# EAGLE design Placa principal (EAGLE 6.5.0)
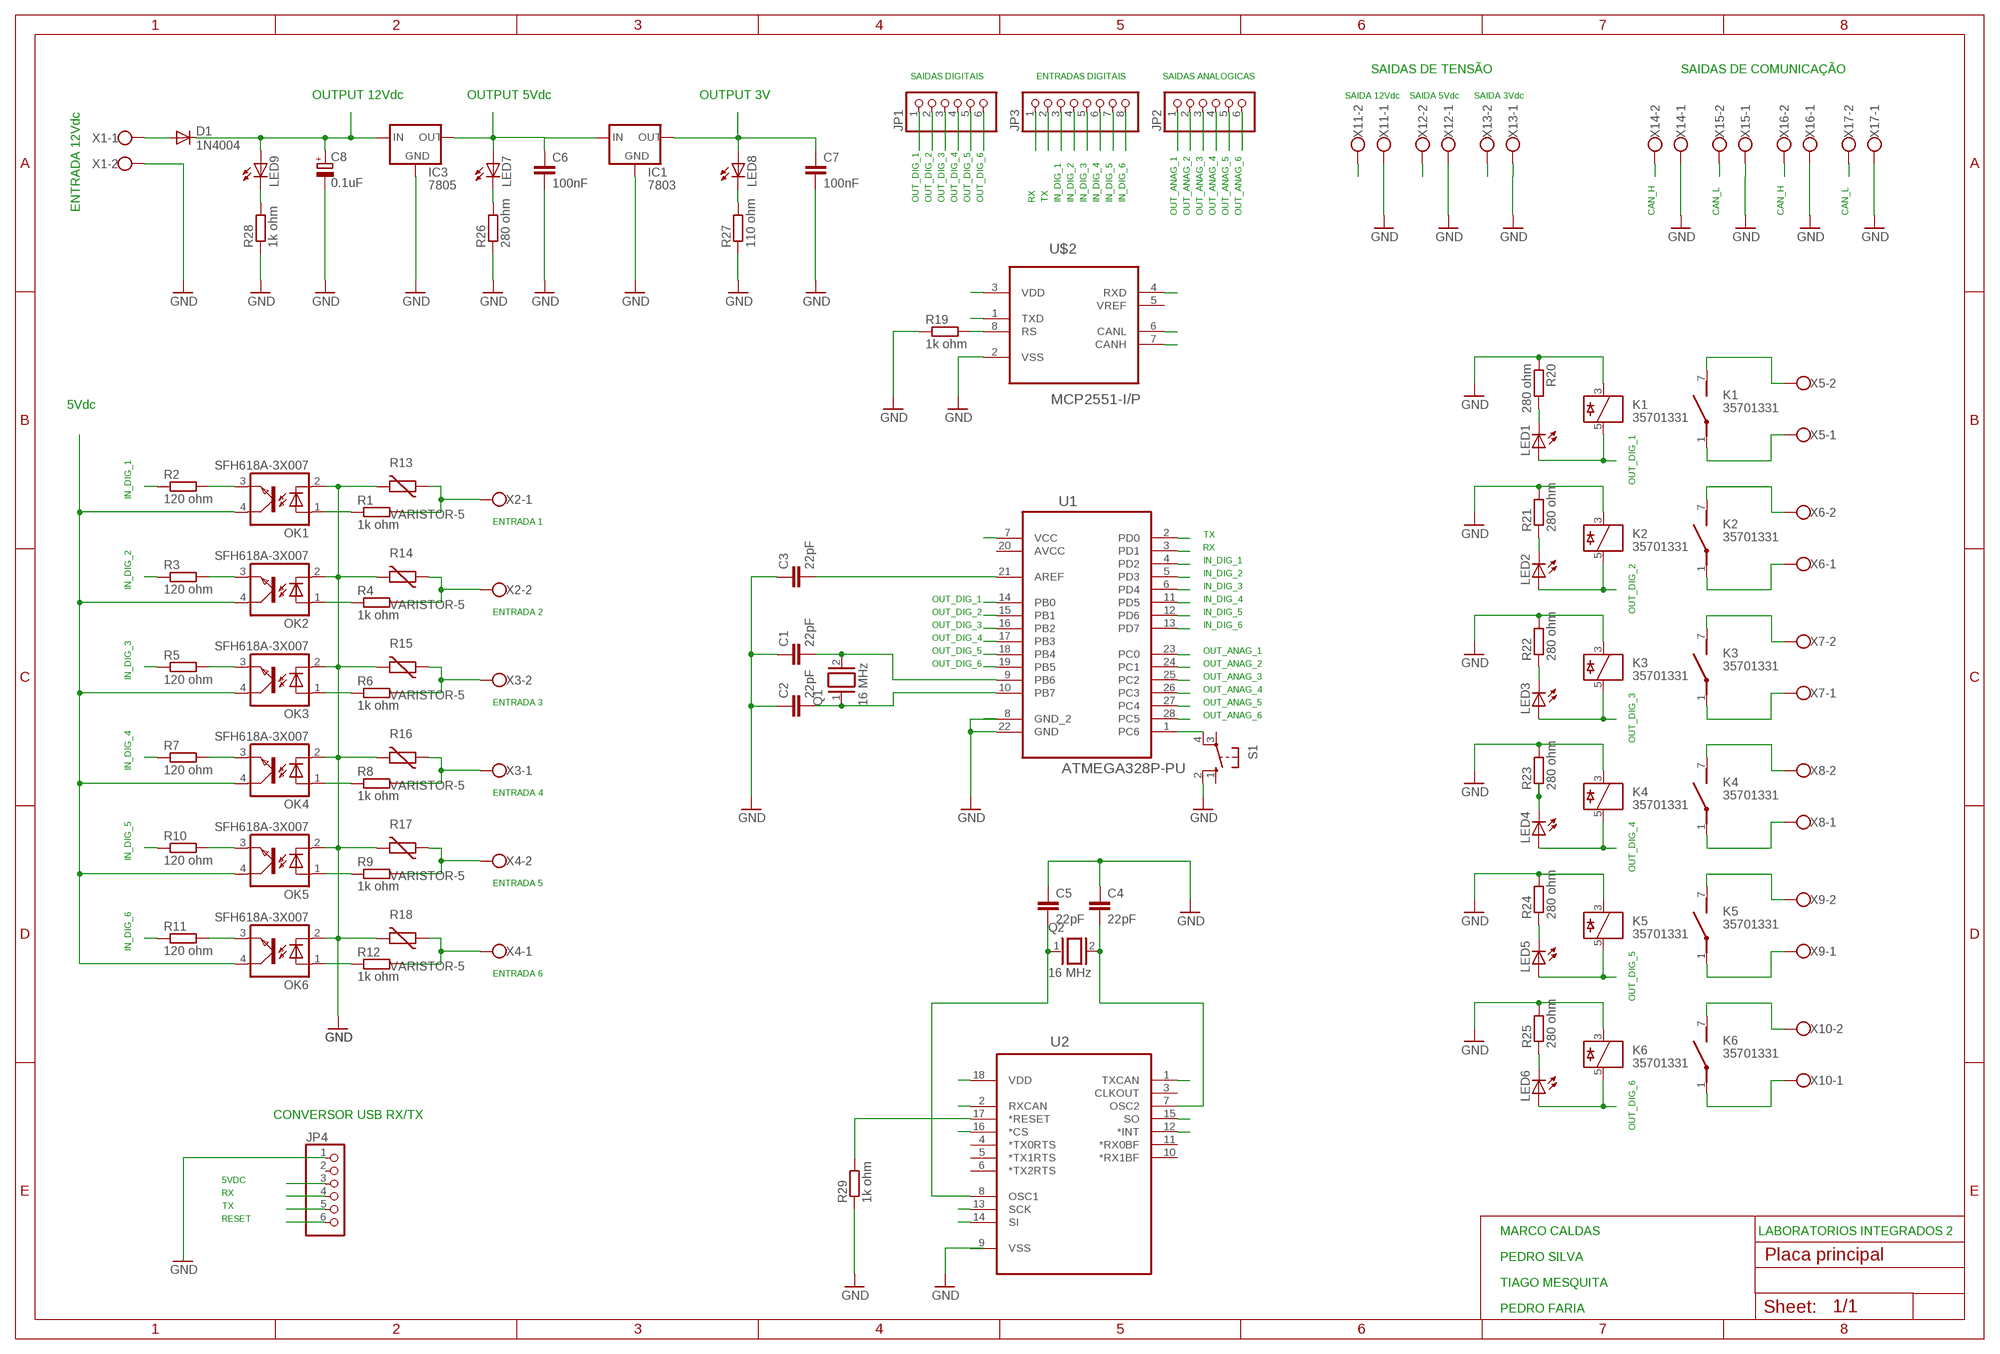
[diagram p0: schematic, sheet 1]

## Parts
C1  22pF  C-EU050-025X075  [C050-025X075]
C2  22pF  C-EU050-025X075  [C050-025X075]
C3  22pF  C-EU050-025X075  [C050-025X075]
C4  22pF  C-EU050-025X075  [C050-025X075]
C5  22pF  C-EU050-025X075  [C050-025X075]
C6  100nF  C-EU050-025X075  [C050-025X075]
C7  100nF  C-EU050-025X075  [C050-025X075]
C8  0.1uF  CPOL-EUE2.5-7  [E2,5-7]
D1  1N4004  [DO41-10]
IC1  7803  78XXS  [78XXS]
IC3  7805  78XXS  [78XXS]
JP1  PINHD-1X6  [1X06]
JP2  PINHD-1X6  [1X06]
JP3  PINHD-1X8  [1X08]
JP4  PINHD-1X6  [1X06]
K1  35701331  [REED]
K2  35701331  [REED]
K3  35701331  [REED]
K4  35701331  [REED]
K5  35701331  [REED]
K6  35701331  [REED]
LED1  LED5MM  [LED5MM]
LED2  LED5MM  [LED5MM]
LED3  LED5MM  [LED5MM]
LED4  LED5MM  [LED5MM]
LED5  LED5MM  [LED5MM]
LED6  LED5MM  [LED5MM]
LED7  LED5MM  [LED5MM]
LED8  LED5MM  [LED5MM]
LED9  LED5MM  [LED5MM]
OK1  SFH618A-3X007  [SMD4-7]
OK2  SFH618A-3X007  [SMD4-7]
OK3  SFH618A-3X007  [SMD4-7]
OK4  SFH618A-3X007  [SMD4-7]
OK5  SFH618A-3X007  [SMD4-7]
OK6  SFH618A-3X007  [SMD4-7]
Q1  16 MHz  XTAL/S  [QS]
Q2  16 MHz  XTAL/S  [QS]
R1  1k ohm  R-EU_0207/10  [0207/10]
R2  120 ohm  R-EU_0207/10  [0207/10]
R3  120 ohm  R-EU_0207/10  [0207/10]
R4  1k ohm  R-EU_0207/10  [0207/10]
R5  120 ohm  R-EU_0207/10  [0207/10]
R6  1k ohm  R-EU_0207/10  [0207/10]
R7  120 ohm  R-EU_0207/10  [0207/10]
R8  1k ohm  R-EU_0207/10  [0207/10]
R9  1k ohm  R-EU_0207/10  [0207/10]
R10  120 ohm  R-EU_0207/10  [0207/10]
R11  120 ohm  R-EU_0207/10  [0207/10]
R12  1k ohm  R-EU_0207/10  [0207/10]
R13  VARISTOR-5  [R-5]
R14  VARISTOR-5  [R-5]
R15  VARISTOR-5  [R-5]
R16  VARISTOR-5  [R-5]
R17  VARISTOR-5  [R-5]
R18  VARISTOR-5  [R-5]
R19  1k ohm  R-EU_0207/10  [0207/10]
R20  280 ohm  R-EU_0207/10  [0207/10]
R21  280 ohm  R-EU_0207/10  [0207/10]
R22  280 ohm  R-EU_0207/10  [0207/10]
R23  280 ohm  R-EU_0207/10  [0207/10]
R24  280 ohm  R-EU_0207/10  [0207/10]
R25  280 ohm  R-EU_0207/10  [0207/10]
R26  280 ohm  R-EU_0207/10  [0207/10]
R27  110 ohm  R-EU_0207/10  [0207/10]
R28  1k ohm  R-EU_0207/10  [0207/10]
R29  1k ohm  R-EU_0207/10  [0207/10]
S1  10-XX  [B3F-10XX]
U1  ATMEGA328P-PU  [DIP254P762X457-28]
U2  MCP2510-I/P.  [DIP254P762X533-18P]
U$2  MCP2551-I/P  [DIP254P762X432-8]
X1  W237-102  [W237-102]
X2  W237-102  [W237-102]
X3  W237-102  [W237-102]
X4  W237-102  [W237-102]
X5  W237-102  [W237-102]
X6  W237-102  [W237-102]
X7  W237-102  [W237-102]
X8  W237-102  [W237-102]
X9  W237-102  [W237-102]
X10  W237-102  [W237-102]
X11  W237-102  [W237-102]
X12  W237-102  [W237-102]
X13  W237-102  [W237-102]
X14  W237-102  [W237-102]
X15  W237-102  [W237-102]
X16  W237-102  [W237-102]
X17  W237-102  [W237-102]

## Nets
3VDC: C7.1 IC1.OUT LED8.A X13.2
5VDC: C6.1 IC1.IN IC3.OUT JP4.3 LED7.A OK1.4(COL) OK2.4(COL) OK3.4(COL) OK4.4(COL) OK5.4(COL) OK6.4(COL) U1.7(VCC) U2.18(VDD) U$2.3(VDD) X12.2
12VDC: C8.+ D1.C IC3.IN LED9.A X11.2
CAN_H: U$2.7(CANH) X14.2 X16.2
CAN_L: U$2.6(CANL) X15.2 X17.2
CAN_RX: U2.1(TXCAN) U$2.4(RXD)
CAN_TX: U2.2(RXCAN) U$2.1(TXD)
GND: C1.1 C2.1 C3.1 C4.1 C5.1 C6.2 C7.2 C8.- IC1.GND IC3.GND JP4.1 K1.3 K2.3 K3.3 K4.3 K5.3 K6.3 OK1.2(C) OK2.2(C) OK3.2(C) OK4.2(C) OK5.2(C) OK6.2(C) R13.2 R14.2 R15.2 R16.2 R17.2 R18.2 R19.1 R20.1 R21.2 R22.2 R23.2 R24.2 R25.2 R26.1 R27.1 R28.1 R29.1 S1.2(S1) U1.8(GND_2) U1.22(GND) U$2.2(VSS) X1.2 X11.1 X12.1 X14.1 X16.1 X17.1
IN_DIG_1: JP3.3 R2.1 U1.4(PD2) U2.12(*INT)
IN_DIG_2: JP3.4 R3.1 U1.5(PD3)
IN_DIG_3: JP3.5 R5.1 U1.6(PD4)
IN_DIG_4: JP3.6 R7.1 U1.11(PD5)
IN_DIG_5: JP3.7 R10.1 U1.12(PD6)
IN_DIG_6: JP3.8 R11.1 U1.13(PD7)
N$1: OK1.3(EMIT) R2.2
N$2: OK1.1(A) R1.1
N$3: X15.1
N$4: K1.7(2:S) X5.2
N$5: OK2.1(A) R4.1
N$6: OK3.1(A) R6.1
N$7: OK4.1(A) R8.1
N$8: OK2.3(EMIT) R3.2
N$9: OK3.3(EMIT) R5.2
N$10: OK4.3(EMIT) R7.2
N$11: OK5.3(EMIT) R10.2
N$12: OK6.3(EMIT) R11.2
N$13: K1.1(2:P) X5.1
N$14: R1.2 R13.1 X2.1
N$15: OK6.1(A) R12.1
N$16: OK5.1(A) R9.1
N$17: R4.2 R14.1 X2.2
N$18: R6.2 R15.1 X3.2
N$19: R8.2 R16.1 X3.1
N$20: R9.2 R17.1 X4.2
N$21: R12.2 R18.1 X4.1
N$22: LED2.K(C) R21.1
N$24: LED1.K(C) R20.2
N$25: C1.2 Q1.2 U1.9(PB6)
N$26: C2.2 Q1.1 U1.10(PB7)
N$27: K2.7(2:S) X6.2
N$28: C3.2 U1.21(AREF)
N$30: LED3.K(C) R22.1
N$31: R19.2 U$2.8(RS)
N$32: D1.A X1.1
N$33: C4.2 Q2.2 U2.7(OSC2)
N$34: C5.2 Q2.1 U2.8(OSC1)
N$35: R29.2 U2.17(*RESET)
N$38: K2.1(2:P) X6.1
N$39: LED4.K(C) R23.1
N$41: K3.7(2:S) X7.2
N$42: LED5.K(C) R24.1
N$43: LED7.K(C) R26.2
N$44: K3.1(2:P) X7.1
N$45: LED6.K(C) R25.1
N$46: LED8.K(C) R27.2
N$47: K4.7(2:S) X8.2
N$48: LED9.K(C) R28.2
N$50: K4.1(2:P) X8.1
N$51: K5.7(2:S) X9.2
N$52: K5.1(2:P) X9.1
N$53: K6.7(2:S) X10.2
N$54: K6.1(2:P) X10.1
N$57: X13.1
OUT_ANAG_1: JP2.1 U1.23(PC0)
OUT_ANAG_2: JP2.2 U1.24(PC1)
OUT_ANAG_3: JP2.3 U1.25(PC2)
OUT_ANAG_4: JP2.4 U1.26(PC3)
OUT_ANAG_5: JP2.5 U1.27(PC4)
OUT_ANAG_6: JP2.6 U1.28(PC5)
OUT_DIG_1: JP1.1 K1.5 LED1.A U1.14(PB0)
OUT_DIG_2: JP1.2 K2.5 LED2.A U1.15(PB1)
OUT_DIG_3: JP1.3 K3.5 LED3.A U1.16(PB2) U2.16(*CS)
OUT_DIG_4: JP1.4 K4.5 LED4.A U1.17(PB3) U2.14(SI)
OUT_DIG_5: JP1.5 K5.5 LED5.A U1.18(PB4) U2.15(SO)
OUT_DIG_6: JP1.6 K6.5 LED6.A U1.19(PB5) U2.13(SCK)
RESET: JP4.6 S1.4(P1) U1.1(PC6)
RX: JP3.1 JP4.4 U1.3(PD1)
TX: JP3.2 JP4.5 U1.2(PD0)
Unconnected: JP4.2 S1.1(S) S1.3(P) U2.3(CLKOUT) U2.4(*TX0RTS) U2.5(*TX1RTS) U2.6(*TX2RTS) U2.10(*RX1BF) U2.11(*RX0BF) U$2.5(VREF)

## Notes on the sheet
- SAIDAS DIGITAIS | ENTRADAS DIGITAIS | SAIDAS ANALOGICAS | SAIDAS DE TENSÃO | SAIDAS DE COMUNICAÇÃO
- OUTPUT 12Vdc | OUTPUT 5Vdc | OUTPUT 3V | SAIDA 12Vdc | SAIDA 5Vdc | SAIDA 3Vdc
- OUT_DIG_1 | OUT_DIG_2 | OUT_DIG_3 | OUT_DIG_4 | OUT_DIG_5 | OUT_DIG_6 | RX | TX | IN_DIG_1 | IN_DIG_2 | IN_DIG_3 | IN_DIG_4 | IN_DIG_5 | IN_DIG_6
- ENTRADA 12Vdc | OUT_ANAG_1 | OUT_ANAG_2 | OUT_ANAG_3 | OUT_ANAG_4 | OUT_ANAG_5 | OUT_ANAG_6 | CAN_H | CAN_L | CAN_H | CAN_L
- 5Vdc
- OUT_DIG_1
- IN_DIG_1
- ENTRADA 1
- TX
- RX
- IN_DIG_1 | OUT_DIG_2
- IN_DIG_2
- IN_DIG_2 | IN_DIG_3
- OUT_DIG_1 | IN_DIG_4
- ENTRADA 2 | OUT_DIG_2 | IN_DIG_5
- OUT_DIG_3 | IN_DIG_6
- OUT_DIG_4
- OUT_DIG_5 | OUT_ANAG_1
- OUT_DIG_6 | OUT_ANAG_2
- IN_DIG_3 | OUT_ANAG_3
- OUT_ANAG_4 | OUT_DIG_3
- ENTRADA 3 | OUT_ANAG_5
- OUT_ANAG_6
- IN_DIG_4
- ENTRADA 4
- OUT_DIG_4
- IN_DIG_5
- ENTRADA 5
- IN_DIG_6 | OUT_DIG_5
- ENTRADA 6
- OUT_DIG_6
- CONVERSOR USB RX/TX
- 5VDC
- RX
- TX
- RESET
- MARCO CALDAS | LABORATORIOS INTEGRADOS 2
- PEDRO SILVA
- TIAGO MESQUITA
- PEDRO FARIA

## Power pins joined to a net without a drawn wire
AVCC: U1.20(AVCC)
VSS: U2.9(VSS)

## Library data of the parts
C1-C7 = rcl:C-EU: CAPACITOR, European symbol
C8 = rcl:CPOL-EU: POLARIZED CAPACITOR, European symbol
D1 = diode:1N4004: DIODE
IC1 IC3 = v-reg:78XXS: VOLTAGE REGULATOR
JP1 JP2 JP4 = pinhead:PINHD-1X6: PIN HEADER
JP3 = pinhead:PINHD-1X8: PIN HEADER
K1-K6 = relay:35701331: RELAY reed, 1 x norm. open with polarity; OC_FARNELL: unknown; OC_NEWARK: unknown
LED1-LED9 = led:LED: LED
OK1-OK6 = optocoupler:SFH618?*: Optocoupler, Phototransistor Output, Low Input Current Source: Data sheet; OC_FARNELL: unknown; OC_NEWARK: unknown
Q1 Q2 = special:XTAL/S: CRYSTAL
R1-R12 R19-R29 = rcl:R-EU_: RESISTOR, European symbol
R13-R18 = varistor:VARISTOR: VARISTOR
S1 = switch-omron:10-XX: OMRON SWITCH; MPN: B3F-1000; OC_FARNELL: 176432; OC_NEWARK: 36M3542
U1 = atmega 328:ATMEGA328P-PU: 8-bit Microcontroller with In-System Programmable Flash; MPN: ATMEGA328P-PU; OC_FARNELL: 1715487; OC_NEWARK: 15R0268; PACKAGE: PDIP-28; SUPPLIER: Atmel
U2 = MCP2510:MCP2510-I/P.: IC, Stand-Alone CAN Controller with SPI Interface, DIP-18; MPN: MCP2510-I/P.; OC_FARNELL: 9758534; OC_NEWARK: 12C1807; PACKAGE: DIP-18; SUPPLIER: Microchip
U$2 = MCP:MCP2551-I/P: High-Speed CAN Transceiver; DESCRIPTION: CAN CTRL; MPN: MCP2551-I/P; OC_FARNELL: 1292240; OC_NEWARK: 61K2947; PACKAGE: PDIP-8; SUPPLIER: Microchip
X1-X17 = con-wago-500:W237-102: WAGO SCREW CLAMP; MPN: 237-102; OC_FARNELL: unknown; OC_NEWARK: 70K9898

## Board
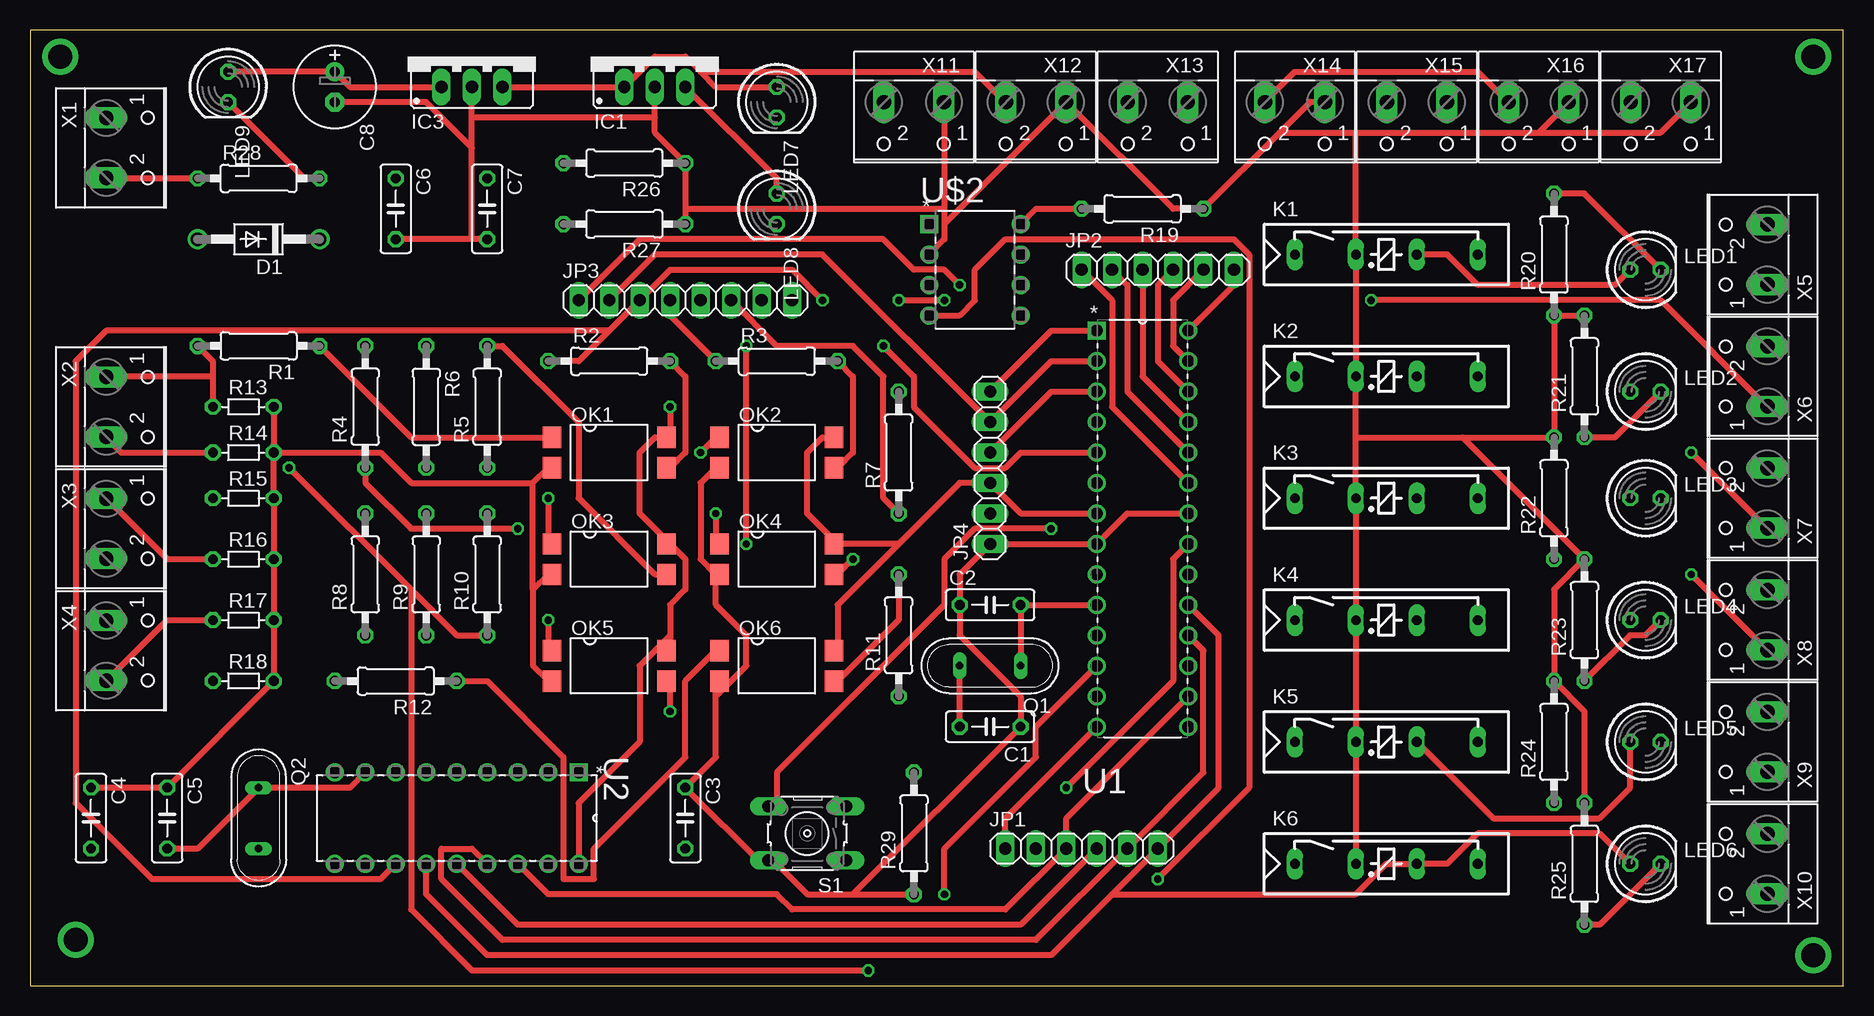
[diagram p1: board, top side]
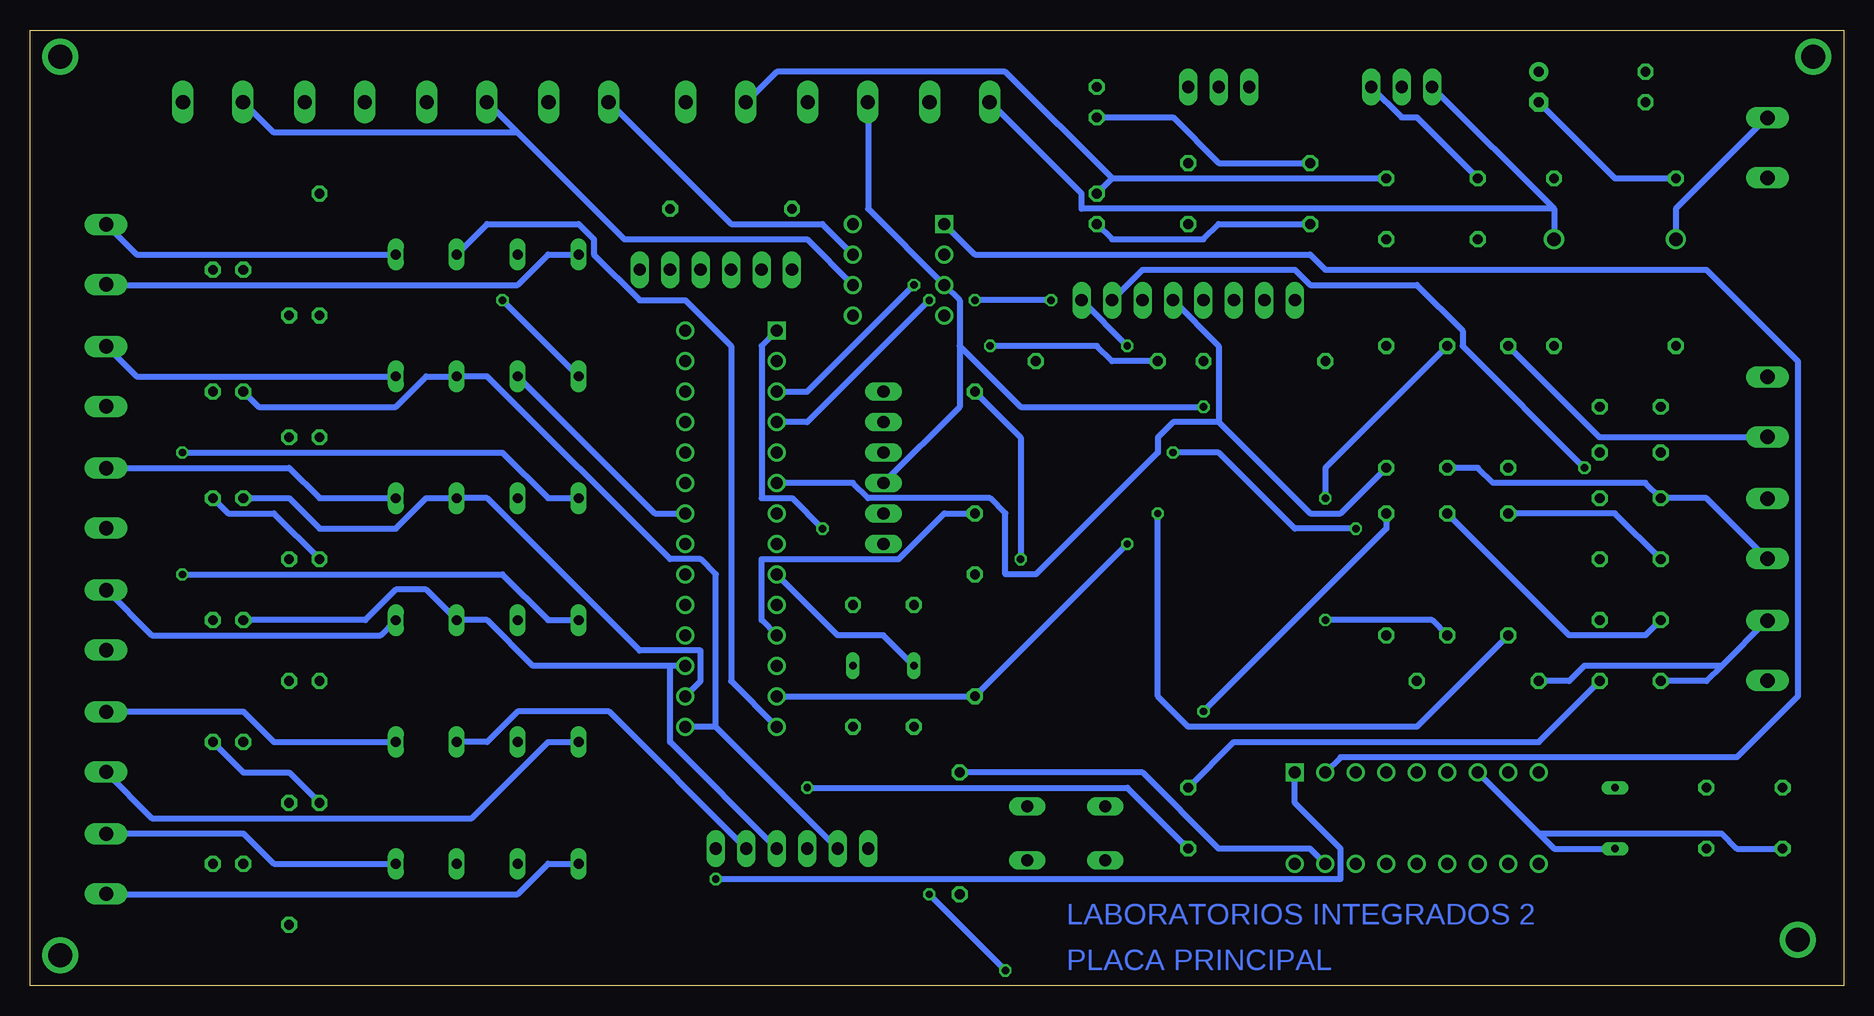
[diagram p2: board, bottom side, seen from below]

Size 151.13 x 79.68 mm. Coordinates in mm from the lower left corner, seen from the top.
Outline: 151.11,0 151.11,79.68 0,79.68 0,0 151.13,0
Copper layers (1*16): Top 0.035mm / dielectric 1.5mm / Bottom 0.035mm
Design rules "default *": minimum track width 20mil, minimum drill 24mil, track to track 16mil, track to pad 8mil, pad to pad 8mil, via to via 16mil, smd to smd 8mil, copper to edge 40mil, drill to drill 8mil, minimum pad ring 10mil, minimum via ring 8mil, stop-mask expansion 4mil, vias tented up to drill 0mil, thermal gap 10mil

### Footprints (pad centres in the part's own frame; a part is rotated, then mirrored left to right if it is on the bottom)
C050-025X075 = drill 0.813 octagon: 1 -2.54,0; 2 2.54,0
E2,5-7 = drill 0.813 pad 1.6: + -1.27,0 | drill 0.813 pad 1.6 octagon: - 1.27,0
DO41-10 = drill 1.118: A 5.08,0; C -5.08,0
78XXS = drill 1.016 long: GND 0,-2.54; IN -2.54,-2.54; OUT 2.54,-2.54
1X06 = drill 1.016 long: 1 -6.35,0; 2 -3.81,0; 3 -1.27,0; 4 1.27,0; 5 3.81,0; 6 6.35,0
1X08 = drill 1.016 long: 1 -8.89,0; 2 -6.35,0; 3 -3.81,0; 4 -1.27,0; 5 1.27,0; 6 3.81,0; 7 6.35,0; 8 8.89,0
REED = drill 0.813 long: 1 -17.78,2.54; 3 -12.7,2.54; 5 -7.62,2.54; 7 -2.54,2.54
LED5MM = drill 0.813 octagon: A -1.27,0; K 1.27,0
SMD4-7 = smd 1.78 x 1.55: 1 -1.27,-4.77; 2 1.27,-4.77; 3 1.27,4.77; 4 -1.27,4.77
QS = drill 0.61 long: 1 -2.54,0; 2 2.54,0
0207/10 = drill 0.813 octagon: 1 -5.08,0; 2 5.08,0
R-5 = drill 0.813 octagon: 1 -2.54,0; 2 2.54,0
B3F-10XX = drill 1.016 long: 1 -3.251,2.261; 2 3.251,2.261; 3 -3.251,-2.261; 4 3.251,-2.261
DIP254P762X457-28 = drill 0.991 square: 1 -7.62,33.02 | drill 0.991: 2 -7.62,30.48; 3 -7.62,27.94; 4 -7.62,25.4; 5 -7.62,22.86; 6 -7.62,20.32; 7 -7.62,17.78; 8 -7.62,15.24; 9 -7.62,12.7; 10 -7.62,10.16; 11 -7.62,7.62; 12 -7.62,5.08; 13 -7.62,2.54; 14 -7.62,0; 15 0,0; 16 0,2.54; 17 0,5.08; 18 0,7.62; 19 0,10.16; 20 0,12.7; 21 0,15.24; 22 0,17.78; 23 0,20.32; 24 0,22.86; 25 0,25.4; 26 0,27.94; 27 0,30.48; 28 0,33.02
DIP254P762X533-18P = drill 0.991 square: 1 -7.62,20.32 | drill 0.991: 2 -7.62,17.78; 3 -7.62,15.24; 4 -7.62,12.7; 5 -7.62,10.16; 6 -7.62,7.62; 7 -7.62,5.08; 8 -7.62,2.54; 9 -7.62,0; 10 0,0; 11 0,2.54; 12 0,5.08; 13 0,7.62; 14 0,10.16; 15 0,12.7; 16 0,15.24; 17 0,17.78; 18 0,20.32
DIP254P762X432-8 = drill 0.991 square: 1 -7.62,7.62 | drill 0.991: 2 -7.62,5.08; 3 -7.62,2.54; 4 -7.62,0; 5 0,0; 6 0,2.54; 7 0,5.08; 8 0,7.62
W237-102 = drill 1.194 long: 1 -2.5,-1.27; 2 2.5,-1.27

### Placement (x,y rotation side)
C1  80.01,21.59 180 top
C2  80.01,31.75 0 top
C3  54.61,13.97 270 top
C4  5.08,13.97 270 top
C5  11.43,13.97 270 top
C6  30.48,64.77 270 top
C7  38.1,64.77 270 top
C8  25.4,74.93 270 top
D1  19.05,62.23 180 top
IC1  52.07,77.47 0 top
IC3  36.83,77.47 0 top
JP1  87.63,11.43 0 top
JP2  93.98,59.69 0 top
JP3  54.61,57.15 0 top
JP4  80.01,43.18 90 top
K1  123.19,58.42 0 top
K2  123.19,48.26 0 top
K3  123.19,38.1 0 top
K4  123.19,27.94 0 top
K5  123.19,17.78 0 top
K6  123.19,7.62 0 top
LED1  134.62,59.69 0 top
LED2  134.62,49.53 0 top
LED3  134.62,40.64 0 top
LED4  134.62,30.48 0 top
LED5  134.62,20.32 0 top
LED6  134.62,10.16 0 top
LED7  62.23,73.66 270 top
LED8  62.23,64.77 270 top
LED9  16.51,74.93 270 top
OK1  48.26,44.45 270 top
OK2  62.23,44.45 270 top
OK3  48.26,35.56 270 top
OK4  62.23,35.56 270 top
OK5  48.26,26.67 270 top
OK6  62.23,26.67 270 top
Q1  80.01,26.67 180 top
Q2  19.05,13.97 270 top
R1  19.05,53.34 180 top
R2  48.26,52.07 0 top
R3  62.23,52.07 0 top
R4  27.94,48.26 90 top
R5  38.1,48.26 90 top
R6  33.02,48.26 270 top
R7  72.39,44.45 90 top
R8  27.94,34.29 90 top
R9  33.02,34.29 90 top
R10  38.1,34.29 90 top
R11  72.39,29.21 90 top
R12  30.48,25.4 180 top
R13  17.78,48.26 0 top
R14  17.78,44.45 0 top
R15  17.78,40.64 0 top
R16  17.78,35.56 0 top
R17  17.78,30.48 0 top
R18  17.78,25.4 0 top
R19  92.71,64.77 180 top
R20  127,60.96 90 top
R21  129.54,50.8 90 top
R22  127,40.64 90 top
R23  129.54,30.48 90 top
R24  127,20.32 90 top
R25  129.54,10.16 90 top
R26  49.53,68.58 180 top
R27  49.53,63.5 180 top
R28  19.05,67.31 0 top
R29  73.66,12.7 90 top
S1  64.77,12.7 180 top
U1  96.52,21.59 0 top
U2  25.4,10.16 270 top
U$2  82.55,55.88 0 top
X1  7.62,69.85 270 top
X2  7.62,48.26 270 top
X3  7.62,38.1 270 top
X4  7.62,27.94 270 top
X5  143.51,60.96 90 top
X6  143.51,50.8 90 top
X7  143.51,40.64 90 top
X8  143.51,30.48 90 top
X9  143.51,20.32 90 top
X10  143.51,10.16 90 top
X11  73.66,72.39 180 top
X12  83.82,72.39 180 top
X13  93.98,72.39 180 top
X14  105.41,72.39 180 top
X15  115.57,72.39 180 top
X16  125.73,72.39 180 top
X17  135.89,72.39 180 top

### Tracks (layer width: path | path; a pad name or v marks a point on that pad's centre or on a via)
3VDC
  Top 0.508: IC1.OUT 62.23,67.31 LED8.A
  Bottom 0.508: 60.96,67.31 C7.1 | LED8.A 60.96,67.31 | 60.96,67.31 69.85,76.2 88.9,76.2 91.44,73.66 X13.2
5VDC  (via drill 0.61)
  Top 0.508: 53.34,29.21 53.34,31.75 54.61,33.02 54.61,35.56 53.34,36.83 | 53.34,29.21 53.34,27.94 OK5.4 | 53.34,36.83 50.8,39.37 50.8,44.45 52.07,45.72 OK1.4 53.34,45.72 v53.34,48.26 | 53.34,36.83 OK3.4 | U2.18 45.72,15.24 50.8,20.32 50.8,26.67 53.34,29.21 | 72.39,36.83 77.47,41.91 JP4.3 82.55,39.37 U1.7 | 72.39,36.83 67.31,31.75 67.31,27.94 OK6.4 | 72.39,36.83 67.31,36.83 | 67.31,36.83 64.77,39.37 64.77,44.45 66.04,45.72 OK2.4 67.31,45.72 | 67.31,36.83 OK4.4 | LED7.A 57.15,74.93 55.88,76.2 | 55.88,76.2 54.61,77.47 52.07,77.47 IC1.IN IC3.OUT | 55.88,76.2 78.74,76.2 81.28,73.66 X12.2
  Bottom 0.508: X12.2 81.28,73.66 81.28,64.77 U$2.3 73.66,57.15 73.66,53.34 | C6.1 35.56,72.39 36.83,72.39 IC3.OUT | JP4.3 73.66,48.26 73.66,53.34 | v53.34,48.26 68.58,48.26 73.66,53.34
12VDC
  Top 0.508: LED9.A C8.+ 26.67,74.93 IC3.IN
  Bottom 0.508: 24.13,64.77 D1.C | IC3.IN 24.13,64.77 | 24.13,64.77 63.5,64.77 63.5,66.04 71.12,73.66 X11.2
CAN_H
  Top 0.508: X16.2 123.19,73.66 120.65,76.2 105.41,76.2 102.87,73.66 X14.2
  Bottom 0.508: U$2.7 85.09,63.5 92.71,63.5 102.87,73.66 X14.2
CAN_L
  Bottom 0.508: U$2.6 86.36,62.23 101.6,62.23 110.49,71.12 | 110.49,71.12 113.03,73.66 X15.2 | 110.49,71.12 130.81,71.12 133.35,73.66 X17.2
CAN_RX  (via drill 0.61)
  Top 0.508: v93.98,8.89 101.6,16.51 101.6,60.96 100.33,62.23 81.28,62.23 78.74,59.69 78.74,57.15 77.47,55.88 U$2.4
  Bottom 0.508: U2.1 45.72,15.24 41.91,11.43 41.91,8.89 v93.98,8.89
CAN_TX
  Bottom 0.508: U2.2 41.91,19.05 8.89,19.05 3.81,24.13 3.81,52.07 11.43,59.69 43.18,59.69 44.45,60.96 72.39,60.96 U$2.1
GND
  Top 0.508: U$2.2 76.2,62.23 76.2,63.5 | 76.2,64.77 76.2,73.66 X11.1 | 76.2,64.77 76.2,63.5 | 76.2,63.5 86.36,73.66 | 54.61,64.77 R26.1 52.07,71.12 52.07,72.39 | 54.61,64.77 R27.1 | 52.07,72.39 IC1.GND | R28.1 6.35,67.31 X1.2 | C7.2 36.83,62.23 | 36.83,62.23 C6.2 | 36.83,62.23 36.83,69.85 | 36.83,69.85 36.83,72.39 | 36.83,72.39 IC3.GND | C8.- 33.02,73.66 36.83,69.85 | 36.83,72.39 52.07,72.39 | 54.61,64.77 76.2,64.77 | 41.91,33.02 41.91,26.67 43.18,25.4 OK5.2 | 41.91,33.02 43.18,34.29 OK3.2 | 41.91,41.91 43.18,43.18 OK1.2 | 41.91,33.02 41.91,41.91 | C4.1 C5.1 R18.2 R17.2 R16.2 R15.2 R14.2 | R13.2 R14.2 | 41.91,41.91 31.75,41.91 29.21,44.45 R14.2 | 57.15,34.29 55.88,35.56 55.88,41.91 57.15,43.18 OK2.2 | 57.15,24.13 57.15,19.05 C3.1 60.96,10.16 S1.2 62.23,10.16 64.77,7.62 68.58,7.62 | 57.15,24.13 57.15,25.4 OK6.2 | 57.15,34.29 57.15,31.75 59.69,29.21 59.69,26.67 57.15,24.13 | 57.15,34.29 OK4.2 | 68.58,7.62 R29.1 | 68.58,7.62 C1.1 82.55,24.13 77.47,29.21 C2.1 77.47,34.29 JP4.1 U1.8 91.44,39.37 U1.22 | 104.14,71.12 106.68,73.66 X14.1 107.95,73.66 | 104.14,71.12 R19.1 95.25,64.77 86.36,73.66 | 125.73,71.12 128.27,73.66 X16.1 | 104.14,71.12 110.49,71.12 | 110.49,71.12 125.73,71.12 | 125.73,71.12 135.89,71.12 138.43,73.66 X17.1 | R25.2 129.54,22.86 R24.2 127,33.02 R23.2 119.38,45.72 | R21.2 R20.1 R22.2 119.38,45.72 | K6.3 K5.3 K4.3 K3.3 110.49,45.72 | 110.49,45.72 K2.3 K1.3 110.49,71.12 | 110.49,45.72 119.38,45.72 | 86.36,73.66 X12.1
  Bottom 0.508: R28.1 19.05,67.31 C8.- | U1.22 99.06,39.37 K2.3 | R18.2 25.4,20.32 50.8,20.32 C3.1
IN_DIG_1  (via drill 0.61)
  Top 0.508: R2.1 45.72,52.07 48.26,54.61 | 48.26,54.61 JP3.3 53.34,59.69 63.5,59.69 v66.04,57.15 | U2.12 29.21,8.89 10.16,8.89 3.81,15.24 3.81,52.07 6.35,54.61 48.26,54.61 | v72.39,57.15 v76.2,57.15
  Bottom 0.508: U1.4 86.36,46.99 v76.2,57.15 | v66.04,57.15 v72.39,57.15
IN_DIG_2  (via drill 0.61)
  Top 0.508: R3.1 53.34,55.88 JP3.4 | U1.5 82.55,44.45 81.28,43.18 78.74,43.18 73.66,48.26 73.66,50.8 v71.12,53.34
  Bottom 0.508: v71.12,53.34 62.23,53.34 60.96,52.07 R3.1
IN_DIG_3
  Bottom 0.508: R5.1 41.91,39.37 44.45,39.37 52.07,46.99 | 52.07,46.99 52.07,53.34 JP3.5 | U1.6 82.55,41.91 81.28,40.64 71.12,40.64 69.85,39.37 69.85,34.29 67.31,34.29 57.15,44.45 57.15,45.72 55.88,46.99 52.07,46.99
IN_DIG_4
  Top 0.508: JP3.6 62.23,53.34 68.58,53.34 71.12,50.8 71.12,40.64 R7.1
  Bottom 0.508: R7.1 74.93,39.37 78.74,35.56 90.17,35.56 90.17,30.48 U1.11
IN_DIG_5  (via drill 0.61)
  Top 0.508: R10.1 35.56,29.21 31.75,33.02 | v21.59,43.18 31.75,33.02 | U1.12 83.82,21.59 83.82,19.05 76.2,11.43 v76.2,7.62 | v69.85,1.27 36.83,1.27 31.75,6.35 31.75,33.02
  Bottom 0.508: v21.59,43.18 31.75,53.34 31.75,54.61 35.56,58.42 44.45,58.42 45.72,59.69 58.42,59.69 JP3.7 | v69.85,1.27 v76.2,7.62
IN_DIG_6  (via drill 0.61)
  Top 0.508: v59.69,36.83 v59.69,53.34
  Bottom 0.508: U1.13 R11.1 v59.69,36.83 | v59.69,53.34 JP3.8
N$1
  Top 0.508: R2.2 54.61,50.8 54.61,44.45 53.34,43.18 OK1.3
N$2
  Top 0.508: OK1.1 31.75,45.72 R1.1
N$4
  Bottom 0.508: K1.7 142.24,60.96 144.78,63.5 X5.2
N$5  (via drill 0.61)
  Top 0.508: v55.88,44.45 57.15,45.72 OK2.1 | v40.64,38.1 31.75,38.1 27.94,41.91 R4.1
  Bottom 0.508: v55.88,44.45 52.07,44.45 45.72,38.1 v40.64,38.1
N$6  (via drill 0.61)
  Top 0.508: v43.18,40.64 43.18,36.83 OK3.1
  Bottom 0.508: v43.18,40.64 43.18,43.18 R6.1
N$7  (via drill 0.61)
  Top 0.508: v57.15,39.37 57.15,36.83 OK4.1
  Bottom 0.508: v57.15,39.37 57.15,24.13 54.61,21.59 35.56,21.59 R8.1
N$8
  Top 0.508: R3.2 68.58,50.8 68.58,44.45 67.31,43.18 OK2.3
N$9
  Top 0.508: R5.2 39.37,53.34 45.72,46.99 45.72,40.64 52.07,34.29 OK3.3 53.34,34.29
N$10  (via drill 0.61)
  Top 0.508: v68.58,35.56 67.31,34.29 OK4.3
  Bottom 0.508: v68.58,35.56 68.58,45.72 R7.2
N$11  (via drill 0.61)
  Top 0.508: v53.34,22.86 53.34,25.4 OK5.3
  Bottom 0.508: v53.34,22.86 38.1,38.1 R10.2
N$12
  Top 0.508: R11.2 72.39,30.48 67.31,25.4 OK6.3
N$13
  Bottom 0.508: K1.1 107.95,60.96 110.49,58.42 144.78,58.42 X5.1
N$14
  Top 0.508: 15.24,50.8 15.24,52.07 R1.2 | 15.24,50.8 R13.1 | 15.24,50.8 6.35,50.8 X2.1
N$15
  Top 0.508: R12.1 38.1,25.4 44.45,19.05 44.45,8.89 46.99,8.89 46.99,11.43 54.61,19.05 54.61,25.4 57.15,27.94 OK6.1
N$16  (via drill 0.61)
  Top 0.508: v43.18,30.48 43.18,27.94 OK5.1
  Bottom 0.508: v43.18,30.48 34.29,30.48 R9.1
N$17
  Top 0.508: R14.1 7.62,44.45 6.35,45.72 X2.2
  Bottom 0.508: R4.2 20.32,45.72 6.35,45.72 X2.2
N$18
  Bottom 0.508: X3.2 6.35,35.56 11.43,40.64 R15.1 16.51,41.91 29.21,41.91 30.48,43.18 R6.2
N$19
  Top 0.508: R16.1 11.43,35.56 6.35,40.64 X3.1
  Bottom 0.508: R8.2 19.05,39.37 R16.1
N$20
  Top 0.508: R17.1 11.43,30.48 6.35,25.4 X4.2
  Bottom 0.508: R9.2 22.86,29.21 16.51,29.21 R17.1
N$21
  Bottom 0.508: R18.1 11.43,25.4 10.16,26.67 | 10.16,26.67 6.35,30.48 X4.1 | R12.2 22.86,25.4 21.59,26.67 10.16,26.67
N$22
  Top 0.508: R21.1 132.08,45.72 LED2.K
N$23  (via drill 2)
  other vias: 148.59,77.47
N$24
  Top 0.508: R20.2 129.54,66.04 LED1.K
N$25
  Top 0.508: C1.2 Q1.2
  Bottom 0.508: U1.9 83.82,29.21 80.01,29.21 Q1.2
N$26
  Top 0.508: Q1.1 C2.2 U1.10
N$27
  Bottom 0.508: K2.7 142.24,50.8 144.78,53.34 X6.2
N$28  (via drill 0.61)
  Top 0.508: v86.36,16.51 95.25,25.4 95.25,35.56 U1.21
  Bottom 0.508: C3.2 59.69,16.51 v86.36,16.51
N$29  (via drill 2)
  other vias: 148.59,2.54
N$30
  Bottom 0.508: R22.1 130.81,39.37 134.62,39.37 LED3.K
N$31
  Top 0.508: R19.2 83.82,64.77 U$2.8
N$32
  Bottom 0.508: D1.A 13.97,64.77 6.35,72.39 X1.1
N$33
  Bottom 0.508: Q2.2 24.13,11.43 25.4,12.7 | U2.7 25.4,12.7 | C4.2 8.89,11.43 10.16,12.7 25.4,12.7
N$34
  Top 0.508: U2.8 26.67,16.51 Q2.1 13.97,11.43 C5.2
N$35
  Bottom 0.508: R29.2 58.42,17.78 52.07,11.43 44.45,11.43 U2.17
N$37  (via drill 2)
  other vias: 3.81,3.81
N$38  (via drill 0.61)
  Top 0.508: v111.76,57.15 135.89,57.15 144.78,48.26 X6.1
  Bottom 0.508: v111.76,57.15 K2.1
N$39
  Top 0.508: R23.1 133.35,29.21 134.62,29.21 LED4.K
N$40  (via drill 2)
  other vias: 2.54,77.47
N$41
  Bottom 0.508: K3.7 127,40.64 129.54,43.18 144.78,43.18 X7.2
N$42
  Bottom 0.508: R24.1 129.54,17.78 133.35,17.78 LED5.K
N$43
  Bottom 0.508: R26.2 52.07,68.58 55.88,72.39 LED7.K
N$44  (via drill 0.61)
  Top 0.508: v138.43,44.45 144.78,38.1 X7.1
  Bottom 0.508: K3.1 107.95,40.64 111.76,44.45 v138.43,44.45
N$45
  Top 0.508: R25.1 130.81,5.08 LED6.K
N$46
  Bottom 0.508: R27.2 52.07,63.5 53.34,62.23 60.96,62.23 LED8.K
N$47
  Bottom 0.508: K4.7 121.92,29.21 140.97,29.21 144.78,33.02 X8.2
N$48
  Top 0.508: LED9.K 22.86,67.31 R28.2
N$50  (via drill 0.61)
  Top 0.508: v138.43,34.29 144.78,27.94 X8.1
  Bottom 0.508: K4.1 107.95,30.48 111.76,34.29 v138.43,34.29
N$51
  Bottom 0.508: K5.7 130.81,20.32 133.35,22.86 144.78,22.86 X9.2
N$52
  Bottom 0.508: K5.1 107.95,20.32 114.3,13.97 140.97,13.97 144.78,17.78 X9.1
N$53
  Bottom 0.508: K6.7 130.81,10.16 133.35,12.7 144.78,12.7 X10.2
N$54
  Bottom 0.508: K6.1 107.95,10.16 110.49,7.62 144.78,7.62 X10.1
OUT_ANAG_1
  Top 0.508: U1.23 90.17,48.26 90.17,57.15 JP2.1
OUT_ANAG_2
  Top 0.508: U1.24 91.44,49.53 91.44,58.42 JP2.2
OUT_ANAG_3
  Top 0.508: U1.25 92.71,50.8 JP2.3
OUT_ANAG_4
  Top 0.508: U1.26 93.98,52.07 93.98,58.42 JP2.4
OUT_ANAG_5
  Top 0.508: U1.27 95.25,53.34 95.25,57.15 JP2.5
OUT_ANAG_6
  Top 0.508: U1.28 100.33,58.42 JP2.6
OUT_DIG_1
  Top 0.508: U1.14 81.28,13.97 JP1.1 | K1.5 118.11,60.96 120.65,58.42 132.08,58.42 LED1.A
  Bottom 0.508: U1.14 92.71,25.4 92.71,53.34 96.52,57.15 100.33,57.15 104.14,60.96 104.14,62.23 105.41,63.5 113.03,63.5 K1.5
OUT_DIG_2
  Bottom 0.508: LED2.A 132.08,48.26 120.65,48.26 118.11,50.8 K2.5 113.03,50.8 97.79,35.56 95.25,35.56 93.98,34.29 93.98,21.59 | 93.98,21.59 U1.15 | JP1.2 93.98,21.59
OUT_DIG_3
  Top 0.508: U2.16 43.18,7.62 62.23,7.62 63.5,6.35 81.28,6.35 JP1.3 86.36,13.97 U1.16
  Bottom 0.508: LED3.A 129.54,40.64 127,38.1 120.65,38.1 118.11,40.64 K3.5 113.03,40.64 100.33,27.94 95.25,27.94 95.25,25.4 U1.16
OUT_DIG_4
  Top 0.508: U2.14 40.64,5.08 82.55,5.08 JP1.4
  Bottom 0.508: U1.17 97.79,26.67 | 97.79,26.67 109.22,26.67 113.03,30.48 K4.5 118.11,33.02 120.65,33.02 123.19,30.48 LED4.A | 97.79,26.67 97.79,20.32 JP1.4
OUT_DIG_5
  Top 0.508: LED5.A 133.35,16.51 130.81,13.97 121.92,13.97 K5.5 | U2.15 36.83,11.43 34.29,11.43 34.29,8.89 39.37,3.81 83.82,3.81 JP1.5 97.79,17.78 97.79,27.94 U1.18
  Bottom 0.508: K5.5 113.03,20.32 110.49,22.86 102.87,22.86 JP1.5
OUT_DIG_6
  Top 0.508: LED6.A 130.81,12.7 120.65,12.7 118.11,10.16 K6.5 113.03,10.16 110.49,7.62 90.17,7.62 | U2.13 33.02,7.62 38.1,2.54 85.09,2.54 90.17,7.62 | 90.17,7.62 JP1.6 99.06,16.51 99.06,29.21 U1.19
RESET  (via drill 0.61)
  Top 0.508: U1.1 85.09,54.61 JP4.6 | v85.09,38.1 78.74,38.1 76.2,35.56 76.2,31.75 62.23,17.78 62.23,15.24 S1.4
  Bottom 0.508: v85.09,38.1 87.63,40.64 90.17,40.64 90.17,53.34 U1.1
RX  (via drill 0.61)
  Top 0.508: U1.3 85.09,49.53 JP4.4 | JP3.1 50.8,62.23 71.12,62.23 73.66,59.69 76.2,59.69 v77.47,58.42
  Bottom 0.508: v77.47,58.42 86.36,49.53 U1.3
TX
  Top 0.508: U1.2 85.09,52.07 JP4.5 66.04,60.96 52.07,60.96 JP3.2

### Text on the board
Bottom: LABORATORIOS INTEGRADOS 2 | PLACA PRINCIPAL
